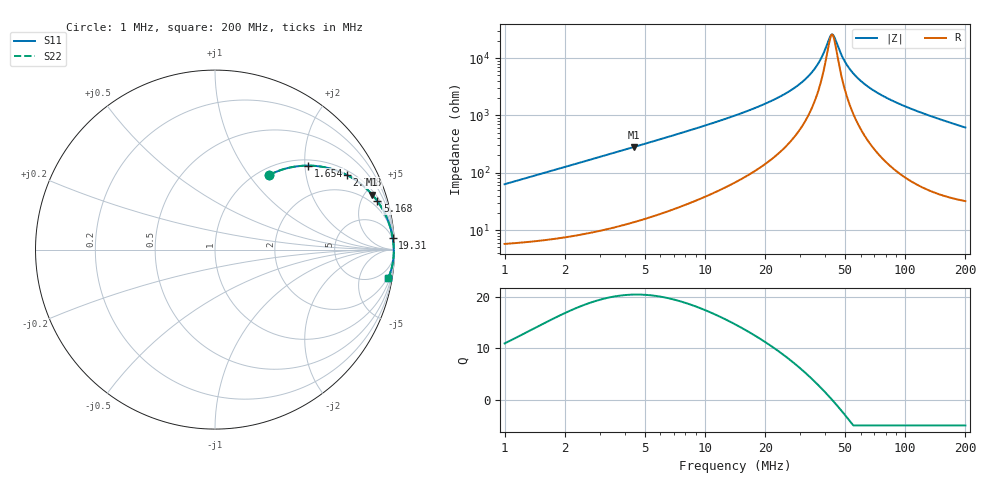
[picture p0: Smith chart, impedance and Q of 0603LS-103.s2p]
# MHz S MA R 50
!Freq  MagS11  AngS11  MagS21  AngS21  MagS12  AngS12  MagS22  AngS22
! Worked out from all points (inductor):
!   801 points, 1 MHz to 200 MHz, reference 50 ohm
!   read as one part in series: L = 10 uH near 1.027 MHz
!   highest Q = 20.4 at 4.438 MHz (marker M1), where L = 10.1 uH
!   self-resonance near 43.03 MHz
!   S11 on the Smith chart (normalised r, x): 1 MHz: 1.11, +1.26; 1.654 MHz: 1.14, +2.08; 2.718 MHz: 1.18, +3.43; 5.168 MHz: 1.32, +6.58; 19.31 MHz: 4, +30; 200 MHz: 2, -12
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1  0.5131 54.1  0.8129 -30.7  0.8129 -30.7  0.5131 54.1
1.654237  0.6993 42.0  0.6706 -44.3  0.6706 -44.3  0.6993 42.0
2.428972  0.8173 32.2  0.5333 -54.7  0.5333 -54.7  0.8173 32.2
2.718438  0.8449 29.4  0.4923 -57.5  0.4923 -57.5  0.8449 29.4
4.437769  0.9283 19.2  0.3293 -68.0  0.3293 -68.0  0.9283 19.2
5.167962  0.9441 16.6  0.2866 -70.6  0.2866 -70.6  0.9441 16.6
5.86096  0.9545 14.7  0.2545 -72.4  0.2545 -72.4  0.9545 14.7
14.14214  0.9883 5.7  0.09945 -80.4  0.09945 -80.4  0.9883 5.7
19.30636  0.9922 3.7  0.06563 -81.3  0.06563 -81.3  0.9922 3.7
27.42482  0.9947 2.0  0.03472 -80.3  0.03472 -80.3  0.9947 2.0
31.10235  0.9953 1.4  0.02486 -78.4  0.02486 -78.4  0.9953 1.4
34.35085  0.9956 1.0  0.01742 -75.0  0.01742 -75.0  0.9956 1.0
37.43943  0.9959 0.6  0.01124 -68.1  0.01124 -68.1  0.9959 0.6
41.90117  0.9961 0.1  0.004469 -28.9  0.004469 -28.9  0.9961 0.1
43.31193  0.9961 -0.0  0.003871 3.9  0.003871 3.9  0.9961 -0.0
44.47467  0.9962 -0.1  0.00442 29.8  0.00442 29.8  0.9962 -0.1
49.77481  0.9962 -0.6  0.01115 70.0  0.01115 70.0  0.9962 -0.6
55.70658  0.9962 -1.1  0.01929 78.1  0.01929 78.1  0.9962 -1.1
65.73758  0.9959 -1.8  0.03202 81.8  0.03202 81.8  0.9959 -1.8
82.88649  0.995 -2.9  0.05147 83.0  0.05147 83.0  0.995 -2.9
120.9016  0.9915 -5.1  0.08942 82.0  0.08942 82.0  0.9915 -5.1
200  0.9789 -9.2  0.1594 77.8  0.1594 77.8  0.9789 -9.2
